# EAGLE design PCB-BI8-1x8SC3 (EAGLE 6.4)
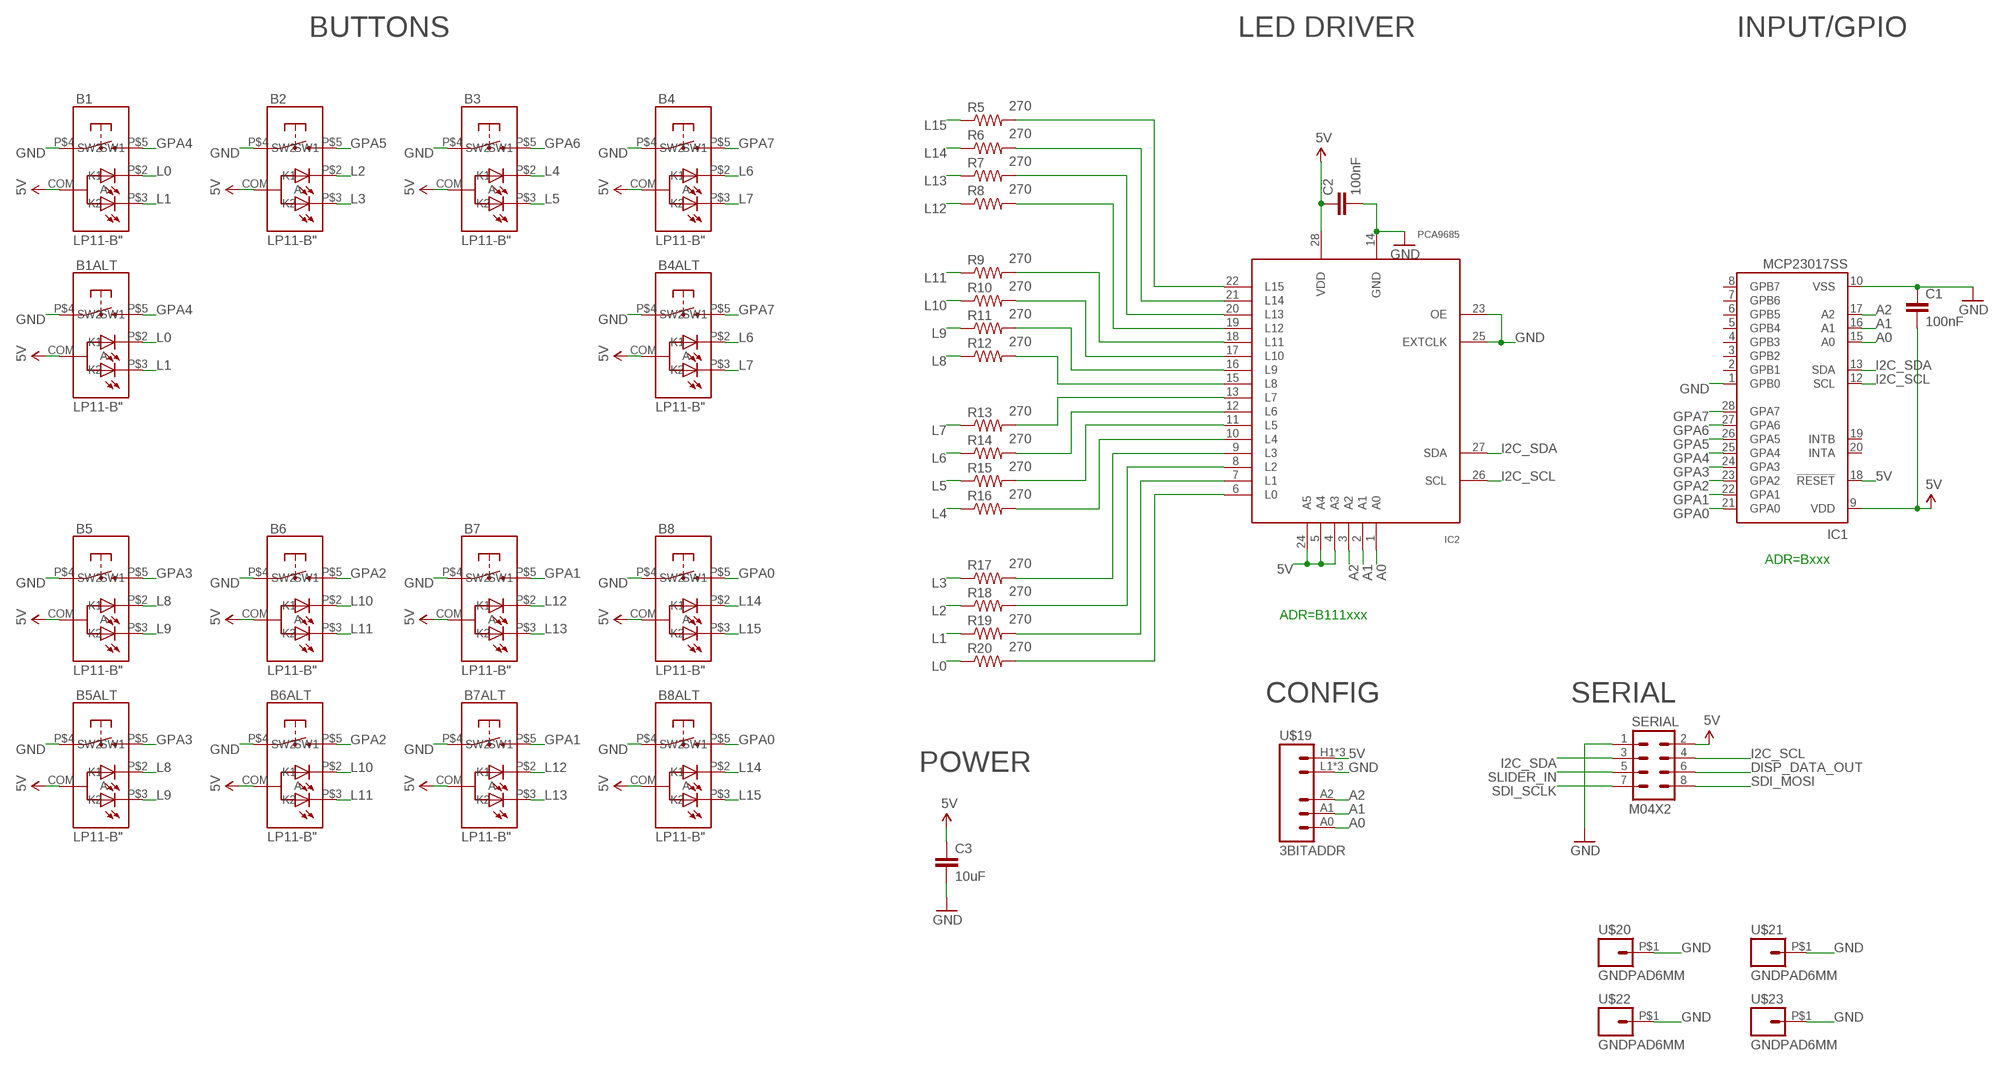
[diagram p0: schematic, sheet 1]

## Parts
B1  LP11-B"  [LP11]
B1ALT  LP11-B"  [LP11]
B2  LP11-B"  [LP11]
B3  LP11-B"  [LP11]
B4  LP11-B"  [LP11]
B4ALT  LP11-B"  [LP11]
B5  LP11-B"  [LP11]
B5ALT  LP11-B"  [LP11]
B6  LP11-B"  [LP11]
B6ALT  LP11-B"  [LP11]
B7  LP11-B"  [LP11]
B7ALT  LP11-B"  [LP11]
B8  LP11-B"  [LP11]
B8ALT  LP11-B"  [LP11]
C1  100nF  CAP0603-CAP  [0603-CAP]
C2  100nF  CAP0603-CAP  [0603-CAP]
C3  10uF  CAP0805  [0805]
IC1  MCP23017SS  [SSOP28]
IC2  PCA9685  [TSSOP28]
R5  270  RESISTOR0603-RES  [0603-RES]
R6  270  RESISTOR0603-RES  [0603-RES]
R7  270  RESISTOR0603-RES  [0603-RES]
R8  270  RESISTOR0603-RES  [0603-RES]
R9  270  RESISTOR0603-RES  [0603-RES]
R10  270  RESISTOR0603-RES  [0603-RES]
R11  270  RESISTOR0603-RES  [0603-RES]
R12  270  RESISTOR0603-RES  [0603-RES]
R13  270  RESISTOR0603-RES  [0603-RES]
R14  270  RESISTOR0603-RES  [0603-RES]
R15  270  RESISTOR0603-RES  [0603-RES]
R16  270  RESISTOR0603-RES  [0603-RES]
R17  270  RESISTOR0603-RES  [0603-RES]
R18  270  RESISTOR0603-RES  [0603-RES]
R19  270  RESISTOR0603-RES  [0603-RES]
R20  270  RESISTOR0603-RES  [0603-RES]
SERIAL  M04X2  [2X4]
U$19  3BITADDR  [3BITADDR]
U$20  GNDPAD6MM  [3.2MMPAD6MM]
U$21  GNDPAD6MM  [3.2MMPAD6MM]
U$22  GNDPAD6MM  [3.2MMPAD6MM]
U$23  GNDPAD6MM  [3.2MMPAD6MM]

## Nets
5V [Power]: B1.COM(A) B1ALT.COM(A) B2.COM(A) B3.COM(A) B4.COM(A) B4ALT.COM(A) B5.COM(A) B5ALT.COM(A) B6.COM(A) B6ALT.COM(A) B7.COM(A) B7ALT.COM(A) B8.COM(A) B8ALT.COM(A) C1.2 C2.1 C3.1 IC1.9(VDD) IC1.18(!RESET) IC2.4(A3) IC2.5(A4) IC2.24(A5) IC2.28(VDD) SERIAL.2 U$19.H1(VCC) U$19.H2(VCC) U$19.H3(VCC)
A0: IC1.15(A0) IC2.1(A0) U$19.A0
A1: IC1.16(A1) IC2.2(A1) U$19.A1
A2: IC1.17(A2) IC2.3(A2) U$19.A2
DISP_DATA_OUT: SERIAL.6
GND [Power]: B1.P$4(SW1) B1ALT.P$4(SW1) B2.P$4(SW1) B3.P$4(SW1) B4.P$4(SW1) B4ALT.P$4(SW1) B5.P$4(SW1) B5ALT.P$4(SW1) B6.P$4(SW1) B6ALT.P$4(SW1) B7.P$4(SW1) B7ALT.P$4(SW1) B8.P$4(SW1) B8ALT.P$4(SW1) C1.1 C2.2 C3.2 IC1.1(GPB0) IC1.10(VSS) IC2.14(GND) IC2.23(OE) IC2.25(EXTCLK) SERIAL.1 U$19.L1(GND) U$19.L2(GND) U$19.L3(GND) U$20.P$1 U$21.P$1 U$22.P$1 U$23.P$1
GPA0: B8.P$5(SW2) B8ALT.P$5(SW2) IC1.21(GPA0)
GPA1: B7.P$5(SW2) B7ALT.P$5(SW2) IC1.22(GPA1)
GPA2: B6.P$5(SW2) B6ALT.P$5(SW2) IC1.23(GPA2)
GPA3: B5.P$5(SW2) B5ALT.P$5(SW2) IC1.24(GPA3)
GPA4: B1.P$5(SW2) B1ALT.P$5(SW2) IC1.25(GPA4)
GPA5: B2.P$5(SW2) IC1.26(GPA5)
GPA6: B3.P$5(SW2) IC1.27(GPA6)
GPA7: B4.P$5(SW2) B4ALT.P$5(SW2) IC1.28(GPA7)
I2C_SCL: IC1.12(SCL) IC2.26(SCL) SERIAL.4
I2C_SDA: IC1.13(SDA) IC2.27(SDA) SERIAL.3
L0: B1.P$2(K1) B1ALT.P$2(K1) R20.1
L1: B1.P$3(K2) B1ALT.P$3(K2) R19.1
L2: B2.P$2(K1) R18.1
L3: B2.P$3(K2) R17.1
L4: B3.P$2(K1) R16.1
L5: B3.P$3(K2) R15.1
L6: B4.P$2(K1) B4ALT.P$2(K1) R14.1
L7: B4.P$3(K2) B4ALT.P$3(K2) R13.1
L8: B5.P$2(K1) B5ALT.P$2(K1) R12.1
L9: B5.P$3(K2) B5ALT.P$3(K2) R11.1
L10: B6.P$2(K1) B6ALT.P$2(K1) R10.1
L11: B6.P$3(K2) B6ALT.P$3(K2) R9.1
L12: B7.P$2(K1) B7ALT.P$2(K1) R8.1
L13: B7.P$3(K2) B7ALT.P$3(K2) R7.1
L14: B8.P$2(K1) B8ALT.P$2(K1) R6.1
L15: B8.P$3(K2) B8ALT.P$3(K2) R5.1
N$4: IC2.13(L7) R13.2
N$5: IC2.12(L6) R14.2
N$7: IC2.11(L5) R15.2
N$9: IC2.10(L4) R16.2
N$10: IC2.9(L3) R17.2
N$11: IC2.8(L2) R18.2
N$12: IC2.7(L1) R19.2
N$19: IC2.6(L0) R20.2
N$20: IC2.15(L8) R12.2
N$21: IC2.16(L9) R11.2
N$22: IC2.17(L10) R10.2
N$23: IC2.18(L11) R9.2
N$24: IC2.19(L12) R8.2
N$25: IC2.20(L13) R7.2
N$26: IC2.21(L14) R6.2
N$27: IC2.22(L15) R5.2
SDI_MOSI: SERIAL.8
SDI_SCLK: SERIAL.7
SLIDER_IN: SERIAL.5
Unconnected: IC1.2(GPB1) IC1.3(GPB2) IC1.4(GPB3) IC1.5(GPB4) IC1.6(GPB5) IC1.7(GPB6) IC1.8(GPB7) IC1.19(INTB) IC1.20(INTA)

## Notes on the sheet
- BUTTONS | LED DRIVER | INPUT/GPIO
- ADR=Bxxx
- ADR=B111xxx
- CONFIG | SERIAL
- POWER

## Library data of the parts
B1 B1ALT B2-B4 B4ALT B5 B5ALT B6 B6ALT B7 B7ALT B8 B8ALT = SKAARHOJ:LP11-B
C1-C3 = SparkFun:CAP: Capacitor
IC1 = microchip:MCP23017: http://ww1.microchip.com/downloads/en/DeviceDoc/21952a.pdf Source: http://ww1.microchip.com/downloads/en/DeviceDoc/21952a.pdf; MF: MICROCHIP; MPN: MCP23017-E/SS; OC_FARNELL: 1467674; OC_NEWARK: 31K2960
IC2 = wsmith:PCA9685
R5-R20 = SparkFun:RESISTOR: Resistor
SERIAL = SparkFun:M04X2
U$19 = SKAARHOJ:3BITADDR
U$20-U$23 = SKAARHOJ:GNDPAD

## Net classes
0 default: width 0.203 mm, drill 0.406 mm, clearance 0.203 mm
1 Power: width 0.406 mm, drill 0.61 mm, clearance 0.203 mm

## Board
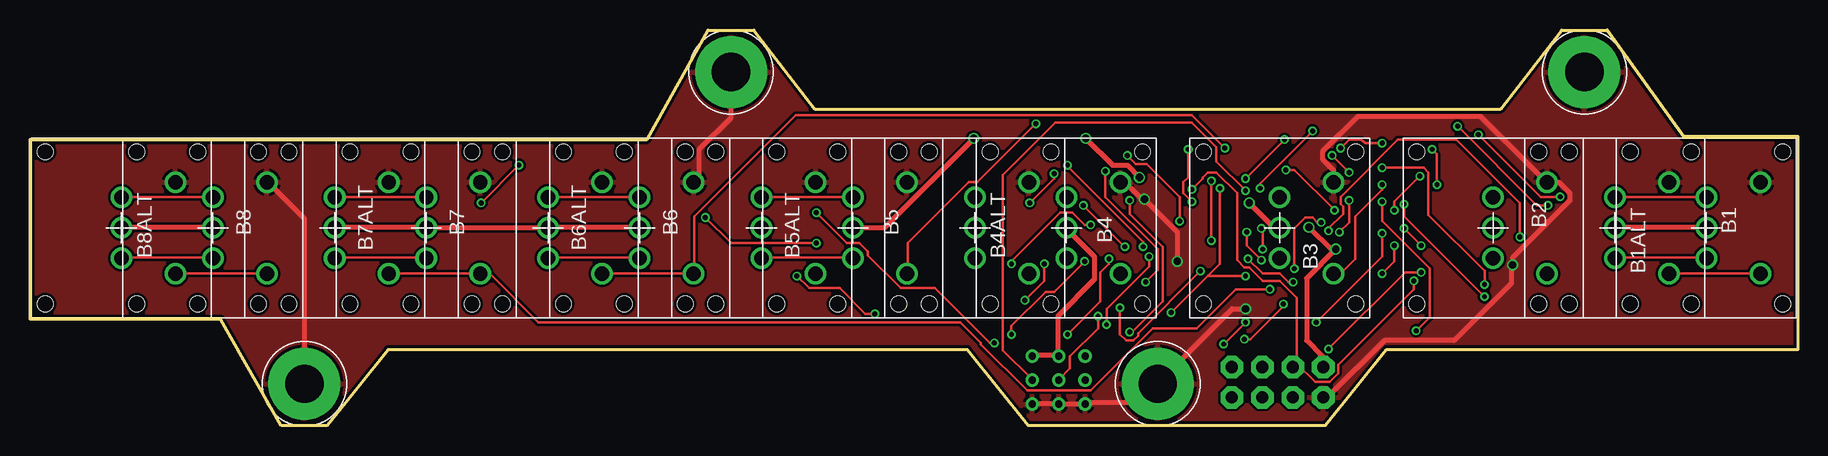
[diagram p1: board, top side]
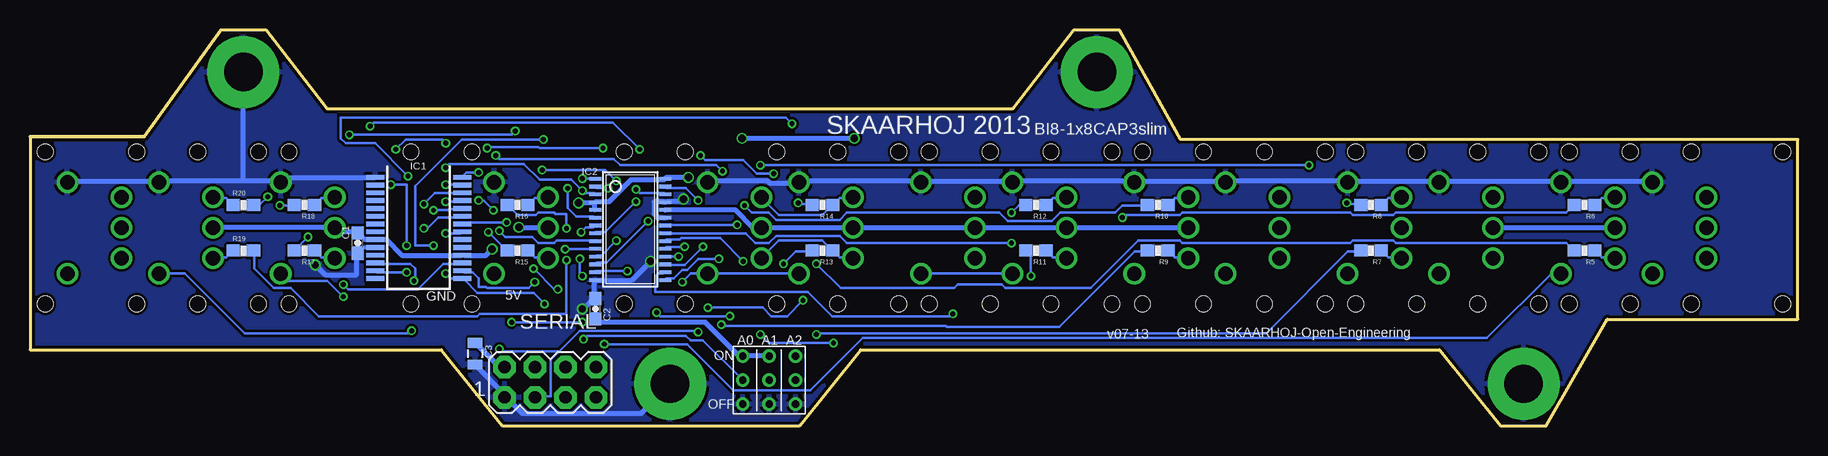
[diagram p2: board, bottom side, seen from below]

Size 147.32 x 33.02 mm. Coordinates in mm from the lower left corner, seen from the top.
Outline: 0,23.88 51.44,23.88 56.52,33.02 60.33,33.02 65.41,26.42 122.56,26.42 127.64,33.02 131.44,33.02 137.79,24.13 147.32,24.13 147.32,6.35 113.03,6.35 107.95,0 83.19,0 78.11,6.35 29.84,6.35 24.77,0 20.95,0 15.88,8.89 0,8.89 0,23.88
Copper layers (1*16): Top 0.035mm / dielectric 1.5mm / Bottom 0.035mm
Design rules "Fusion_eagle_rule_v1.1": minimum track width 6mil, minimum drill 12mil, track to track 6mil, track to pad 6mil, pad to pad 6mil, via to via 6mil, smd to smd 0mil, copper to edge 10mil, drill to drill 10mil, minimum pad ring 10mil, minimum via ring 6mil, stop-mask expansion 2mil, vias tented up to drill 100mil, thermal gap 10mil

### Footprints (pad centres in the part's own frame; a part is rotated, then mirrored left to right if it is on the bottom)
LP11 = drill 1.2: COM 0,0; P$2 0,2.54; P$3 0,-2.54; P$4 4.5,3.81; P$5 4.5,-3.81 | hole 1.3: -6.35,6.35; 6.35,6.35; 6.35,-6.35; -6.35,-6.35
0603-CAP = smd 1.1 x 1: 1 -0.85,0; 2 0.85,0
0805 = smd 0.8 x 1.2: 1 -0.9,0; 2 0.9,0
SSOP28 = smd 0.4 x 1.5: 1 -4.225,-3.625; 2 -3.575,-3.625; 3 -2.925,-3.625; 4 -2.275,-3.625; 5 -1.625,-3.625; 6 -0.975,-3.625; 7 -0.325,-3.625; 8 0.325,-3.625; 9 0.975,-3.625; 10 1.625,-3.625; 11 2.275,-3.625; 12 2.925,-3.625; 13 3.575,-3.625; 14 4.225,-3.625; 15 4.225,3.625; 16 3.575,3.625; 17 2.925,3.625; 18 2.275,3.625; 19 1.625,3.625; 20 0.975,3.625; 21 0.325,3.625; 22 -0.325,3.625; 23 -0.975,3.625; 24 -1.625,3.625; 25 -2.275,3.625; 26 -2.925,3.625; 27 -3.575,3.625; 28 -4.225,3.625
TSSOP28 = smd 0.305 x 0.991: 1 -4.225,-2.918; 2 -3.575,-2.918; 3 -2.925,-2.918; 4 -2.275,-2.918; 5 -1.625,-2.918; 6 -0.975,-2.918; 7 -0.325,-2.918; 8 0.325,-2.918; 9 0.975,-2.918; 10 1.625,-2.918; 11 2.275,-2.918; 12 2.925,-2.918; 13 3.575,-2.918; 14 4.225,-2.918; 15 4.225,2.918; 16 3.575,2.918; 17 2.925,2.918; 18 2.275,2.918; 19 1.625,2.918; 20 0.975,2.918; 21 0.325,2.918; 22 -0.325,2.918; 23 -0.975,2.918; 24 -1.625,2.918; 25 -2.275,2.918; 26 -2.925,2.918; 27 -3.575,2.918; 28 -4.225,2.918
0603-RES = smd 1.1 x 1: 1 -0.85,0; 2 0.85,0
2X4 = drill 1.016 pad 1.88 octagon: 1 -3.81,-1.27; 2 -3.81,1.27; 3 -1.27,-1.27; 4 -1.27,1.27; 5 1.27,-1.27; 6 1.27,1.27; 7 3.81,-1.27; 8 3.81,1.27
3BITADDR = drill 0.6: A0 -2.2,0; A1 0,0; A2 2.2,0; H1 -2.2,2; H2 0,2; H3 2.2,2; L1 -2.2,-2; L2 0,-2; L3 2.2,-2
3.2MMPAD6MM = drill 3.2 pad 6: P$1 0,0

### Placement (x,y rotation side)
B1  139.7,16.51 0 top
B1ALT  132.08,16.51 0 top
B2  121.92,16.51 0 top
B3  104.14,16.51 0 top
B4  86.36,16.51 0 top
B4ALT  78.74,16.51 0 top
B5  68.58,16.51 0 top
B5ALT  60.96,16.51 0 top
B6  50.8,16.51 0 top
B6ALT  43.18,16.51 0 top
B7  33.02,16.51 0 top
B7ALT  25.4,16.51 0 top
B8  15.24,16.51 0 top
B8ALT  7.62,16.51 0 top
C1  120.02,15.24 90 bottom
C2  100.2,9.75 90 bottom
C3  110.24,6.02 270 bottom
IC1  114.94,16.51 270 bottom
IC2  97.31,16.38 270 bottom
R5  17.78,14.61 180 bottom
R6  17.78,18.41 180 bottom
R7  35.56,14.61 180 bottom
R8  35.56,18.41 180 bottom
R9  53.34,14.61 180 bottom
R10  53.34,18.41 180 bottom
R11  63.5,14.61 180 bottom
R12  63.5,18.41 180 bottom
R13  81.28,14.61 180 bottom
R14  81.28,18.41 180 bottom
R15  106.68,14.61 180 bottom
R16  106.68,18.41 180 bottom
R17  124.46,14.61 180 bottom
R18  124.46,18.41 180 bottom
R19  129.54,14.61 0 bottom
R20  129.54,18.41 0 bottom
SERIAL  103.96,3.63 0 bottom
U$19  85.72,3.81 0 bottom
U$20  22.86,3.5 0 top
U$21  93.98,3.5 0 top
U$22  129.54,29.52 0 top
U$23  58.42,29.52 0 top

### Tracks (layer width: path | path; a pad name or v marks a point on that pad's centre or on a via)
5V  (via drill 0.61)
  Top 0.406: v101.6,18.59 103.63,16.56 104.14,16.56 B3.COM | B1ALT.COM 132.08,16.56 139.7,16.56 B1.COM | SERIAL.2 107.7,4.98 107.7,5.79 106.38,7.11 106.38,12.29 v108.81,14.73 108.51,14.63 v106.58,16.56 | B6.COM 50.8,16.56 43.18,16.56 B6ALT.COM 43.08,16.56 33.12,16.56 B7.COM 33.02,16.56 25.4,16.56 B7ALT.COM | B8ALT.COM 7.62,16.56 15.24,16.56 B8.COM | U$19.H3 83.62,5.89 85.65,5.89 U$19.H2 85.65,6.1 85.65,9.14 88.7,12.19 88.7,14.12 86.36,16.46 B4.COM | v92.46,20.73 91.44,21.74 90.22,21.74 v87.99,23.98 | v78.64,23.98 71.22,16.56 68.58,16.56 B5.COM
  Bottom 0.406: IC2.5 100.28,18.09 100.28,18.59 IC2.4 | IC2.4 100.08,18.69 99.06,18.69 97.23,20.52 94.49,20.52 IC2.28 94.28,20.73 v92.46,20.73 | v101.6,18.59 100.48,18.59 IC2.4 | C3.1 108.31,4.98 107.8,4.98 SERIAL.2 | v108.81,14.73 109.32,14.22 111.15,14.22 IC1.18 111.35,14.22 116.33,14.22 117.65,15.54 118.36,15.54 IC1.9 119.48,15.54 119.99,16.05 C1.2 120.19,16.15 121.61,16.15 121.92,16.46 B2.COM 122.02,16.56 132.08,16.56 B1ALT.COM | v106.58,16.56 104.14,16.56 B3.COM | B8.COM 15.24,16.56 25.4,16.56 B7ALT.COM | C2.1 100.18,8.84 99.97,8.64 91.03,8.64 88.29,5.89 87.99,5.89 U$19.H1 87.78,5.89 85.75,5.89 U$19.H2 | IC2.24 94.39,17.98 88.49,17.98 87.07,16.56 86.36,16.56 B4.COM 86.26,16.56 78.74,16.56 B4ALT.COM 78.64,16.56 68.68,16.56 B5.COM 68.58,16.56 60.96,16.56 B5ALT.COM 60.86,16.56 50.8,16.56 B6.COM | v78.64,23.98 v87.99,23.98
A0  (via drill 0.41)
  Top 0.203: v104.55,23.88 v101.3,20.62 | v113.69,15.04 113.69,13.72 v112.67,12.7 | v101.19,7.21 101.7,7.21 104.44,9.96 v104.44,10.16
  Bottom 0.203: v101.3,20.62 100.28,20.62 IC2.1 | v104.55,23.88 111.35,23.88 115.21,20.02 115.21,15.04 v113.69,15.04 | v112.67,12.7 112.27,12.29 111.35,12.29 IC1.15 111.25,12.19 111.15,12.19 110.03,11.07 105.36,11.07 v104.44,10.16 | v101.19,7.21 100.89,7.52 92.66,7.52 92.25,7.11 91.24,7.11 87.99,3.86 U$19.A0
A1  (via drill 0.41)
  Top 0.203: v99.16,19.81 99.16,13.51 98.2,12.55 | v95.1,9.45 98.2,12.55 | v89,9.14 89,8.13 86.67,5.79 86.67,4.78 85.75,3.86 U$19.A1 | v105.26,11.99 104.85,11.99 104.14,12.7 102.72,12.7 v101.5,13.92 | v101.3,12.5 98.25,12.5 98.2,12.55
  Bottom 0.203: v99.16,19.81 100.08,19.81 100.18,19.91 IC2.2 | v95.1,9.45 94.79,9.14 v89,9.14 | v105.26,11.99 105.77,11.48 109.22,11.48 109.32,11.58 109.93,11.58 109.93,12.29 110.44,12.8 111.15,12.8 111.25,12.9 IC1.16 | v101.5,13.92 101.5,12.5 v101.3,12.5
A2  (via drill 0.41)
  Top 0.203: v101.3,19.61 98.86,22.05 98.86,23.27 96.83,25.3 85.45,25.3 81.08,20.93 81.08,6.3 83.52,3.86 U$19.A2 | v121.21,11.79 121.21,12.9 116.53,17.58 116.53,21.13 116.13,21.54 v112.67,21.54
  Bottom 0.203: IC2.3 100.28,19.41 101.09,19.41 v101.3,19.61 102.21,20.52 104.85,20.52 106.17,21.84 112.37,21.84 v112.67,21.54 | v121.21,11.79 120.8,11.38 115.01,11.38 112.88,13.51 111.35,13.51 IC1.17
GND  (via drill 0.61)
  Top 0.406: U$19.L3 83.62,1.83 85.65,1.83 U$19.L2 85.85,1.83 87.88,1.83 U$19.L1 88.09,1.93 92.46,1.93 93.88,3.35 U$21.P$1 93.98,3.56 100.18,9.75 v101.3,9.75 | B3.P$4 108.61,20.32 108.61,21.34 107.7,22.25 107.7,22.86 110.64,25.81 120.9,25.81 126.29,20.42 B2.P$4 127.41,20.32 128.32,19.41 128.32,18.8 123.55,14.02 v123.55,13.41 123.44,13.31 123.44,11.89 118.67,7.11 112.88,7.11 108.2,2.44 107.8,2.44 SERIAL.1 | B4.P$4 91.24,20.32 92.66,18.9 v92.86,18.9 95.61,16.15 v95.61,13.72 | U$20.P$1 22.86,17.27 19.81,20.32 B8.P$4 | U$23.P$1 58.42,25.7 55.78,23.06 55.78,20.73 55.37,20.32 B6.P$4
  Bottom 0.305: IC1.10 120.02,14.88 C1.1
  Bottom 0.406: C3.2 110.24,5.08 107.8,2.64 107.8,2.44 SERIAL.1 107.59,2.34 106.27,1.02 96.42,1.02 93.98,3.45 U$21.P$1 | v101.3,9.75 101.19,9.75 100.38,10.57 C2.2 100.28,10.67 100.28,12.09 IC2.14 100.08,12.09 97.23,12.09 v95.61,13.72 | B1.P$4 144.17,20.32 144.07,20.42 136.75,20.42 136.65,20.32 B1ALT.P$4 136.45,20.42 129.54,20.42 | v123.55,13.41 122.73,12.6 120.09,12.6 120.09,14.33 C1.1 | IC1.1 125.98,20.73 126.39,20.32 B2.P$4 126.59,20.42 129.54,20.42 | 129.54,20.42 U$22.P$1 | IC2.23 94.49,17.37 95,17.37 95.3,17.68 95.3,18.69 94.49,18.69 IC2.25 94.18,18.69 93.07,18.69 v92.86,18.9 | B4.P$4 90.83,20.32 90.73,20.42 85.85,20.42 85.65,20.22 83.41,20.22 B4ALT.P$4 83.21,20.32 83.11,20.42 73.25,20.42 B5.P$4 73.05,20.32 72.95,20.42 65.63,20.42 65.53,20.32 B5ALT.P$4 65.33,20.42 55.47,20.42 B6.P$4 55.27,20.32 55.17,20.42 47.85,20.42 47.75,20.32 B6ALT.P$4 47.55,20.42 37.69,20.42 B7.P$4 37.49,20.32 37.39,20.42 30.07,20.42 29.97,20.32 B7ALT.P$4 29.77,20.42 19.91,20.42 B8.P$4 19.71,20.32 19.61,20.42 12.29,20.42 12.19,20.32 B8ALT.P$4
  pour Top: 0,0 147.32,0 147.32,33.02 0,33.02
  pour Bottom: 0,0 147.32,0 147.32,33.02 0,33.02
GPA0  (via drill 0.41)
  Top 0.203: v112.67,16.05 112.67,14.12 v107.19,8.64 | v99.47,6.81 v101.3,8.64 | B8.P$5 B8ALT.P$5
  Bottom 0.203: v112.67,16.05 111.45,16.05 111.35,16.15 IC1.21 | v101.3,8.64 v107.19,8.64 | v99.47,6.81 92.56,6.81 88.7,2.95 82.3,2.95 77.93,7.32 25.91,7.32 20.52,12.7 B8.P$5
GPA1  (via drill 0.41)
  Top 0.203: v107.59,16.97 107.29,16.97 106.88,17.37 106.27,17.37 105.36,16.46 v105.36,13.11 | v103.33,11.38 100.48,11.38 97.23,8.13 93.57,8.13 88.39,2.95 83.11,2.95 79.25,6.81 79.25,6.91 77.52,8.64 42.37,8.64 38.3,12.7 B7.P$5 B7ALT.P$5
  Bottom 0.203: v107.59,16.97 111.15,16.97 111.25,16.87 IC1.22 | v105.36,13.11 103.63,11.38 v103.33,11.38
GPA2  (via drill 0.41)
  Top 0.203: v115.93,15.04 v114.5,16.46 | v117.25,20.12 117.25,22.66 v116.84,23.06 | v112.67,23.57 111.25,23.57 110.95,23.88 109.93,23.88 v109.22,23.16 | v99.57,23.16 96.83,25.91 63.8,25.91 55.37,17.48 55.37,12.7 B6.P$5 B6ALT.P$5
  Bottom 0.203: v114.5,16.46 114.2,16.46 113.28,17.37 111.45,17.37 111.35,17.48 IC1.23 | v115.93,15.04 115.93,20.12 v117.25,20.12 | v116.84,23.06 116.03,23.88 112.98,23.88 v112.67,23.57 | v109.22,23.16 109.12,23.27 104.95,23.27 104.85,23.16 v99.57,23.16
GPA3  (via drill 0.41)
  Top 0.203: v113.69,17.98 113.69,18.69 v115.82,20.83 | v83.82,25.2 78.94,20.32 78.23,20.32 73.15,15.24 73.15,12.7 B5.P$5
  Bottom 0.203: v113.69,17.98 112.37,17.98 112.27,18.09 111.35,18.09 IC1.24 | v115.82,20.83 118.57,23.57 121.01,23.57 121.41,23.98 121.41,25.7 84.33,25.7 v83.82,25.2 | B5.P$5 B5ALT.P$5
GPA4  (via drill 0.41)
  Top 0.203: v112.67,18.69 112.67,17.07 116.64,13.11 116.64,9.04 v115.52,7.92 | B1ALT.P$5 B1.P$5
  Bottom 0.203: v112.67,18.69 111.35,18.69 IC1.25 | v115.52,7.92 115.72,7.72 129.44,7.72 134.42,12.7 B1ALT.P$5
GPA5  (via drill 0.41)
  Top 0.203: v114.5,18.49 114.5,17.48 v121.21,10.77
  Bottom 0.203: v114.5,18.49 113.59,19.41 111.35,19.41 IC1.26 | v121.21,10.77 122.53,12.09 125.78,12.09 126.39,12.7 B2.P$5
GPA6  (via drill 0.41)
  Top 0.203: v112.67,20.12 112.67,19.71 110.44,17.48 110.44,13.92 109.22,12.7 B3.P$5
  Bottom 0.203: v112.67,20.12 111.35,20.12 IC1.27
GPA7  (via drill 0.41)
  Top 0.203: v108.51,22.55 v109.93,21.13 | v89.61,21.23 89.61,19.1 93.98,14.73 93.98,13.01 v92.96,11.99
  Bottom 0.203: v109.93,21.13 110.95,21.13 111.25,20.83 IC1.28 | v108.51,22.55 108.2,22.25 98.65,22.25 98.15,21.74 90.12,21.74 v89.61,21.23 | v92.96,11.99 92.25,12.7 B4.P$5 B4ALT.P$5
I2C_SCL  (via drill 0.41)
  Top 0.203: v96.83,19.71 97.74,20.62 97.74,20.73 98.15,21.13 98.86,21.13 100.58,19.41 100.58,13.82 101.19,13.21 101.6,13.21 102.72,12.09 104.14,12.09 105.56,10.67 105.56,5.28 105.26,4.98 SERIAL.4 105.56,5.18 107.09,3.66 108.31,3.66 109.02,4.37 109.02,5.08 115.32,11.38 v115.32,12.09
  Bottom 0.203: v96.83,19.71 96.52,19.41 94.49,19.41 IC2.26 | v115.32,12.09 115.21,12.09 115.21,13.11 115.62,13.51 118.47,13.51 IC1.12
I2C_SDA  (via drill 0.41)
  Top 0.203: v91.64,18.8 91.64,17.68 94.39,14.94 94.39,10.36 91.85,7.82 v91.64,7.82 | v115.93,12.8 114.61,12.8 v108.2,6.4
  Bottom 0.203: v91.64,18.8 92.66,19.81 94.28,19.81 94.39,19.91 IC2.27 | v91.64,7.82 91.75,7.92 101.5,7.92 103.28,6.15 | 103.28,6.15 103.94,5.49 103.94,2.44 105.16,2.44 SERIAL.3 | v115.93,12.8 118.36,12.8 118.47,12.9 IC1.13 | v108.2,6.4 108,6.2 103.33,6.2 103.28,6.15
L0
  Top 0.203: B1ALT.P$2 132.08,19.1 139.7,19.1 B1.P$2
  Bottom 0.203: R20.1 130.45,18.49 130.96,19 132.08,19 B1ALT.P$2
L1
  Top 0.203: B1ALT.P$3 132.08,14.02 139.7,14.02 B1.P$3
  Bottom 0.203: R19.1 130.45,14.53 130.96,14.02 132.08,14.02 B1ALT.P$3
L2
  Bottom 0.203: R18.1 123.55,18.49 123.04,19 121.92,19 B2.P$2
L3
  Bottom 0.203: R17.1 123.55,14.53 123.04,14.02 121.92,14.02 B2.P$3
L4
  Bottom 0.203: R16.1 105.77,18.49 105.26,19 104.14,19 B3.P$2
L5
  Bottom 0.203: R15.1 105.77,14.53 105.26,14.02 104.14,14.02 B3.P$3
L6
  Bottom 0.203: B4ALT.P$2 78.74,19 79.86,19 80.37,18.49 R14.1 80.47,18.39 81.28,17.58 84.94,17.58 86.36,19 B4.P$2
L7
  Bottom 0.203: B4ALT.P$3 78.74,14.02 79.86,14.02 80.37,14.53 R13.1 80.47,14.63 81.28,15.44 84.94,15.44 86.36,14.02 B4.P$3
L8
  Top 0.203: B5ALT.P$2 60.96,19.1 68.58,19.1 B5.P$2
  Bottom 0.203: R12.1 62.59,18.49 62.08,19 60.96,19 B5ALT.P$2
L9
  Top 0.203: B5ALT.P$3 60.96,14.02 68.58,14.02 B5.P$3
  Bottom 0.203: R11.1 62.59,14.53 62.08,14.02 60.96,14.02 B5ALT.P$3
L10
  Top 0.203: B6ALT.P$2 43.18,19.1 50.8,19.1 B6.P$2
  Bottom 0.203: R10.1 52.43,18.49 51.92,19 50.8,19 B6.P$2
L11
  Top 0.203: B6ALT.P$3 43.18,14.02 50.8,14.02 B6.P$3
  Bottom 0.203: R9.1 52.43,14.53 51.92,14.02 50.8,14.02 B6.P$3
L12
  Top 0.203: B7ALT.P$2 25.4,19.1 33.02,19.1 B7.P$2
  Bottom 0.203: R8.1 34.65,18.49 34.14,19 33.02,19 B7.P$2
L13
  Top 0.203: B7ALT.P$3 25.4,14.02 33.02,14.02 B7.P$3
  Bottom 0.203: R7.1 34.65,14.53 34.14,14.02 33.02,14.02 B7.P$3
L14
  Top 0.203: B8ALT.P$2 7.62,19.1 15.24,19.1 B8.P$2
  Bottom 0.203: R6.1 16.87,18.49 16.36,19 15.24,19 B8.P$2
L15
  Top 0.203: B8ALT.P$3 7.62,14.02 15.24,14.02 B8.P$3
  Bottom 0.203: R5.1 16.87,14.53 16.36,14.02 15.24,14.02 B8.P$3
N$4  (via drill 0.41)
  Top 0.203: v97.54,12.9 92.35,7.72 92.35,7.52 91.95,7.11 91.34,7.11 90.83,7.62 v90.83,9.86 | v82.91,10.46 84.53,12.09 v84.53,13.51
  Bottom 0.203: v97.54,12.9 100.18,12.9 IC2.13 | v90.83,9.86 86.26,9.86 85.55,9.14 84.23,9.14 v82.91,10.46 | v84.53,13.51 83.52,14.53 82.19,14.53 R13.2
N$5  (via drill 0.41)
  Top 0.203: v95.81,17.07 95.81,19.1 93.07,21.84 92.15,21.84 v91.44,22.55 | v85.34,21.03 85.34,20.62 v83.31,18.59
  Bottom 0.203: v95.81,17.07 99.26,13.61 100.08,13.61 100.18,13.51 IC2.12 | v91.44,22.55 91.03,22.15 87.88,22.15 86.77,21.03 v85.34,21.03 | v83.31,18.59 83.21,18.49 82.19,18.49 R14.2
N$7  (via drill 0.41)
  Top 0.203: v98.45,20.42 v98.45,15.44 | v104.65,21.34 105.36,21.34 v108.71,17.98 | v109.93,18.8 109.93,16.97 v109.12,16.15
  Bottom 0.203: v98.45,15.44 99.67,14.22 100.08,14.22 100.18,14.12 IC2.11 | v98.45,20.42 99.36,21.34 v104.65,21.34 | v108.71,17.98 109.53,18.8 v109.93,18.8 | v109.12,16.15 107.59,14.63 R15.2
N$9  (via drill 0.41)
  Top 0.203: v102.72,14.73 102.72,16.36 v102.62,16.46
  Bottom 0.203: v102.72,14.73 100.28,14.73 IC2.10 | v102.62,16.46 102.62,17.68 103.53,17.68 103.63,17.78 104.95,17.78 105.16,17.58 106.68,17.58 107.49,18.39 R16.2
N$10  (via drill 0.41)
  Top 0.203: v108.2,16.26 108.2,16.46 109.42,17.68 109.42,18.29 109.22,18.49 109.22,19.1 114,23.88 118.87,23.88 124.16,18.59 v124.16,15.75
  Bottom 0.203: v108.2,16.26 107.7,15.75 105.46,15.75 104.95,15.24 103.63,15.24 103.43,15.44 100.28,15.44 IC2.9 | v124.16,15.75 125.27,14.63 R17.2
N$11  (via drill 0.41)
  Top 0.203: v96.83,18.69 96.11,19.41 96.11,20.32 96.52,20.73 v96.52,23.06 | v118.97,24.99 125.58,18.39 v126.49,18.39
  Bottom 0.203: v96.83,18.69 99.36,16.15 100.18,16.15 IC2.8 | v96.52,23.06 98.75,25.3 118.67,25.3 v118.97,24.99 | v126.49,18.39 125.37,18.39 R18.2
N$12  (via drill 0.41)
  Top 0.203: v101.4,16.15 101.4,15.04 v102.62,13.82
  Bottom 0.203: v101.4,16.15 100.99,16.56 100.38,16.56 100.28,16.66 IC2.7 | v102.62,13.82 102.62,9.35 109.83,9.35 110.03,9.14 123.24,9.14 125.58,11.48 127,11.48 128.63,13.11 128.63,14.53 R19.2
N$19  (via drill 0.41)
  Top 0.203: v102.51,19.81 102.51,20.22 v106.88,24.59 | v120.7,24.28 125.88,19.1 v127.51,19.1
  Bottom 0.203: v102.51,19.81 102.51,18.19 101.8,17.48 100.38,17.48 100.28,17.37 IC2.6 | v106.88,24.59 107.19,24.28 v120.7,24.28 | v127.51,19.1 128.12,18.49 128.63,18.49 R20.2
N$20  (via drill 0.41)
  Top 0.203: v89.92,13.92 89.92,13.51 89.2,12.8 89.2,10.36 v86.46,7.62 | v80.37,6.91 79.96,6.91 75.39,11.48 72.54,11.48 69.8,14.22 69.8,14.53 69.09,15.24 68.07,15.24 v65.53,17.78
  Bottom 0.203: v89.92,13.92 91.64,13.92 92.56,13.01 92.96,13.01 93.67,12.29 94.28,12.29 94.39,12.19 IC2.15 | v86.46,7.62 85.75,6.91 v80.37,6.91 | v65.53,17.78 64.92,18.39 64.41,18.39 R12.2
N$21  (via drill 0.41)
  Top 0.203: v70.41,9.35 69.6,9.35 67.46,11.48 64.92,11.48 v63.91,12.5
  Bottom 0.203: v70.41,9.35 70.61,9.14 80.47,9.14 82.5,11.18 95.2,11.18 95.2,12.5 95,12.7 94.59,12.7 94.49,12.8 IC2.16 | v63.91,12.5 63.91,14.53 64.31,14.53 R11.2
N$22  (via drill 0.41)
  Top 0.203: v87.78,18.39 v91.24,14.94
  Bottom 0.203: v91.24,14.94 92.76,13.41 94.39,13.41 IC2.17 | v87.78,18.39 87.17,17.78 85.75,17.78 85.14,17.17 79.86,17.17 79.25,17.78 66.55,17.78 65.84,17.07 62.18,17.07 61.47,17.78 56.9,17.78 56.29,18.39 54.25,18.39 R10.2
N$23  (via drill 0.41)
  Top 0.203: v93.27,14.12 93.27,13.31 89.71,9.75 v89.71,8.43
  Bottom 0.203: v93.27,14.12 94.39,14.12 IC2.18 | v89.71,8.43 89.61,8.33 71.02,8.33 70.92,8.23 61.57,8.23 55.27,14.53 54.25,14.53 R9.2
N$24  (via drill 0.41)
  Top 0.203: v92.76,14.94 92.76,15.34 86.46,21.64 v86.46,21.74 | v37.59,18.59 v40.74,21.74
  Bottom 0.203: v92.76,14.94 94.28,14.94 94.39,14.83 IC2.19 | v40.74,21.74 v86.46,21.74 | v37.59,18.59 37.49,18.49 36.47,18.49 R8.2
N$25  (via drill 0.41)
  Top 0.203: v87.88,13.72 85.34,11.18 84.63,11.18 81.79,8.33 v81.79,7.62
  Bottom 0.203: v87.88,13.72 89.81,15.65 93.07,15.65 93.17,15.54 94.28,15.54 94.39,15.44 IC2.20 | v81.79,7.62 81.69,7.72 44.3,7.72 37.49,14.53 36.47,14.53 R7.2
N$26  (via drill 0.41)
  Top 0.203: v65.53,15.24 58.42,15.24 v56.29,17.37
  Bottom 0.203: v65.53,15.24 79.25,15.24 79.86,15.85 85.14,15.85 85.75,15.24 86.87,15.24 87.68,16.05 IC2.21 | v56.29,17.37 56.08,17.58 51.51,17.58 51.31,17.78 37.29,17.78 37.08,17.58 33.73,17.58 33.53,17.78 19.3,17.78 18.69,18.39 R6.2
N$27  (via drill 0.41)
  Top 0.203: v88.39,16.76 87.88,16.76 86.87,17.78 85.85,17.78 81.79,13.72 v81.79,13.51
  Bottom 0.203: v88.39,16.76 94.39,16.76 IC2.22 | v81.79,13.51 79.76,11.48 70.31,11.48 70,11.79 66.34,11.79 66.04,11.48 58.93,11.48 54.97,15.44 51.51,15.44 51.31,15.24 37.29,15.24 37.08,15.44 33.73,15.44 33.53,15.24 19.3,15.24 18.69,14.63 R5.2

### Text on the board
_bsilk: BI8-1x8CAP3slim | SKAARHOJ 2013 | GND | 5V | v07-13 | Github: SKAARHOJ-Open-Engineering | 1

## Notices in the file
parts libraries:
SparkFun: Licensing: CC v3.0 Share-Alike You are welcome to use this library for commercial purposes.
